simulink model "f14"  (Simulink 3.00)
settings: Solver=ode45  SolverMode=SingleTasking  StartTime=0.0  StopTime=60  RelTol=1e-4  AbsTol=1e-6
PreLoadFcn:
  | f14dat
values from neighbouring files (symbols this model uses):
  a = figure('Color',[0.8 0.8 0.8],     'Position',[25 45 560 420],     'IntegerHandle','off',     'Number','off',    'Name','ÈÎÒâÐÎÊ½×ø±êÑÝÊ¾',    'Tag','Aspectzcx')    [arzcx.m]    (also in f14dat.m = 2.5348; f14def.m = 2.5348; rss.m = zeros([n n arraydims]); watergui.m = 1-str2num(get_param('water/Flush Pulse/PulseConst','value')))
  b = uicontrol('Parent',a,     'Unit',StdUnit,     'BackgroundColor',StdColor,     'Position',PointsPerPixel*[24 28 497 20],     'Units','Normalized',    'Style','text',    'String','Ä¬ÈÏ3DÊÓÍ¼',    'Tag','StatusText')    [arzcx.m]    (also in f14dat.m = 64.13; f14def.m = 64.13; rss.m = b .* (bnz+repmat(zerob,[n m])))
  g = 32.18    [absdata.m]    (also in f14dat.m = 32.2; watergui.m = locdrawwater(hilim, lolim, inflow, outflow, area); watersfun.m = get(ax,'UserData'))
  Ka = 0.6770    (= 0.677)    [f14dat.m]    (also in f14def.m)
  Kf = 1    [absdata.m]    (also in f14dat.m = -1.746; f14def.m = -1.746)
  Ki = -3.8640    (= -3.864)    [f14dat.m]    (also in f14def.m)
  Kq = 0.8156    [f14dat.m]    (also in f14def.m)
  Md = -6.8847    [f14dat.m]    (also in f14def.m)
  Mq = -0.6571    [f14dat.m]    (also in f14def.m)
  Mw = -0.00592    [f14dat.m]    (also in f14def.m)
  Swg = 3    [f14dat.m]    (also in f14def.m)
  Ta = 0.0500    (= 0.05)    [f14dat.m]    (also in f14def.m)
  Tal = 0.3959    [f14dat.m]    (also in f14def.m)
  Ts = 0.1000    (= 0.1)    [f14dat.m]    (also in f14def.m)
  Uo = 689.4000    (= 689.4)    [f14dat.m]    (also in f14def.m)
  Vto = 690.4000    (= 690.4)    [f14dat.m]    (also in f14def.m)
  W1 = 2.9710    (= 2.971)    [f14dat.m]    (also in f14def.m)
  W2 = 4.1440    (= 4.144)    [f14dat.m]    (also in f14def.m)
  Zd = -63.9979    [f14dat.m]    (also in f14def.m)
  Zw = -0.6385    [f14dat.m]    (also in f14def.m)
libraries: simulink x1

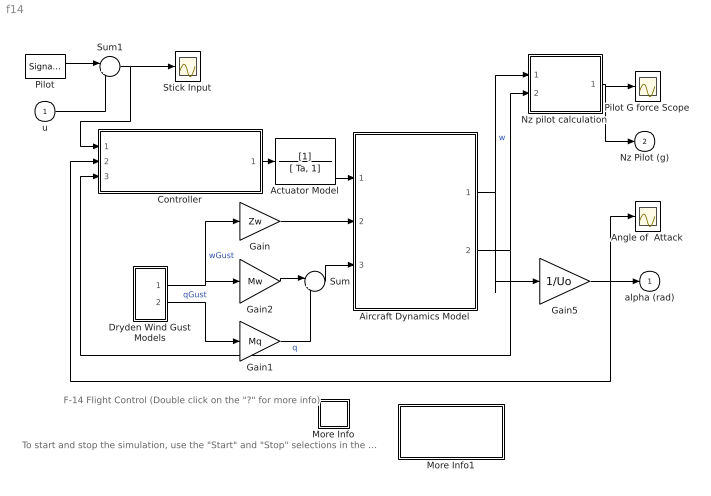
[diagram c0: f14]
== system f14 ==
  note: To start and stop the simulation, use the "Start" and "Stop" selections in the "Simulation" pull-down menu.
  note: F-14 Flight Control (Double click on the "?" for more info)
  u : Inport  Port=1  PortWidth=-1  SampleTime=-1  DataType=auto
  Actuator Model : TransferFcn  Numerator=[1]  Denominator=[ Ta, 1]
  Aircraft Dynamics Model : Subsystem
  Angle of  Attack : Scope
  Controller : Subsystem
  Dryden Wind Gust Models : Subsystem
  Gain : Gain  Gain=Zw  SaturateOnIntegerOverflow=on
  Gain1 : Gain  Gain=Mq  SaturateOnIntegerOverflow=on
  Gain2 : Gain  Gain=Mw  SaturateOnIntegerOverflow=on
  Gain5 : Gain  Gain=1/Uo  SaturateOnIntegerOverflow=on
  More Info : Subsystem
  More Info1 : Subsystem
  Nz pilot calculation : Subsystem
  Pilot : SignalGenerator  WaveForm=square  Amplitude=1  Frequency=0.500000  Units=rad/sec
  Pilot G force Scope : Scope
  Stick Input : Scope
  Sum : Sum  Inputs=|++  SaturateOnIntegerOverflow=on
  Sum1 : Sum  Inputs=|++  SaturateOnIntegerOverflow=on
  alpha (rad) : Outport  Port=1  InitialOutput=0
  Nz Pilot (g) : Outport  Port=2  InitialOutput=0
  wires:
  Gain5/1 -> alpha (rad)/1, Angle of  Attack/1, Controller/2(alpha (rad))
  Aircraft Dynamics Model/1(Vertical Velocity w (ft/sec)) -> Gain5/1, Nz pilot calculation/1(w)  "w"
  Nz pilot calculation/1(Pilot g force (g)) -> Pilot G force Scope/1, Nz Pilot (g)/1
  Gain2/1 -> Sum/1
  Gain/1 -> Aircraft Dynamics Model/2(Vertical Gust wGust (ft/sec))
  Pilot/1 -> Sum1/1
  u/1 -> Sum1/2
  Dryden Wind Gust Models/2(Qg) -> Gain1/1  "qGust"
  Dryden Wind Gust Models/1(Wg) -> Gain2/1, Gain/1  "wGust"
  Sum/1 -> Aircraft Dynamics Model/3(Rotary Gust qGust (rad/sec))
  Gain1/1 -> Sum/2
  Aircraft Dynamics Model/2(Pitch Rate q (rad/sec)) -> Nz pilot calculation/2(q), Controller/3(q (rad/sec))  "q"
  Actuator Model/1 -> Aircraft Dynamics Model/1(Elevator Deflection d (deg))
  Controller/1(Elevator Command (deg)) -> Actuator Model/1
  Sum1/1 -> Stick Input/1, Controller/1(Stick Input (in))

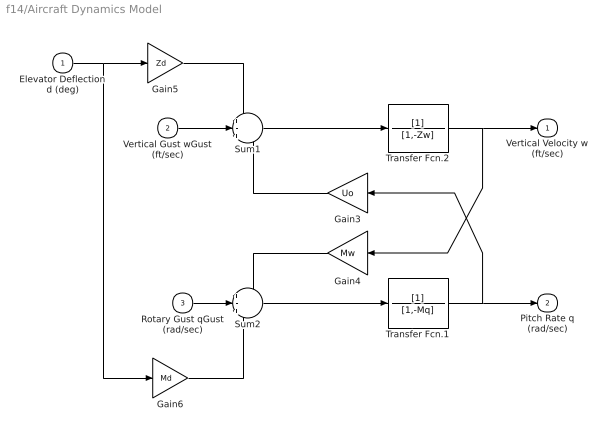
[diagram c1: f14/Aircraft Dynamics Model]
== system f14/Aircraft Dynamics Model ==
  Elevator Deflection d (deg) : Inport  Port=1  PortWidth=-1  SampleTime=-1  DataType=auto
  Vertical Gust wGust (ft/sec) : Inport  Port=2  PortWidth=-1  SampleTime=-1  DataType=auto
  Rotary Gust qGust (rad/sec) : Inport  Port=3  PortWidth=-1  SampleTime=-1  DataType=auto
  Gain3 : Gain  Orientation=left  Gain=Uo  SaturateOnIntegerOverflow=on
  Gain4 : Gain  Orientation=left  Gain=Mw  SaturateOnIntegerOverflow=on
  Gain5 : Gain  Gain=Zd  SaturateOnIntegerOverflow=on
  Gain6 : Gain  Gain=Md  SaturateOnIntegerOverflow=on
  Sum1 : Sum  Inputs=+-+  SaturateOnIntegerOverflow=on
  Sum2 : Sum  Inputs=+-+  SaturateOnIntegerOverflow=on
  Transfer Fcn.1 : TransferFcn  Numerator=[1]  Denominator=[1,-Mq]
  Transfer Fcn.2 : TransferFcn  Numerator=[1]  Denominator=[1,-Zw]
  Vertical Velocity w (ft/sec) : Outport  Port=1  InitialOutput=0
  Pitch Rate q (rad/sec) : Outport  Port=2  InitialOutput=0
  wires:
  Transfer Fcn.2/1 -> Vertical Velocity w (ft/sec)/1, Gain4/1
  Transfer Fcn.1/1 -> Pitch Rate q (rad/sec)/1, Gain3/1
  Gain6/1 -> Sum2/3
  Gain5/1 -> Sum1/1
  Gain3/1 -> Sum1/3
  Rotary Gust qGust (rad/sec)/1 -> Sum2/2
  Sum2/1 -> Transfer Fcn.1/1
  Sum1/1 -> Transfer Fcn.2/1
  Gain4/1 -> Sum2/1
  Vertical Gust wGust (ft/sec)/1 -> Sum1/2
  Elevator Deflection d (deg)/1 -> Gain5/1, Gain6/1

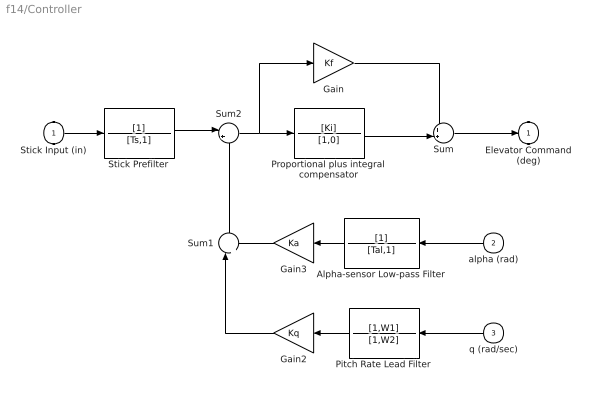
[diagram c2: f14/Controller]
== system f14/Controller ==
  Stick Input (in) : Inport  Port=1  PortWidth=-1  SampleTime=-1  DataType=auto
  alpha (rad) : Inport  Orientation=left  Port=2  PortWidth=-1  SampleTime=-1  DataType=auto
  q (rad/sec) : Inport  Orientation=left  Port=3  PortWidth=-1  SampleTime=-1  DataType=auto
  Alpha-sensor Low-pass Filter : TransferFcn  Orientation=left  Numerator=[1]  Denominator=[Tal,1]
  Gain : Gain  Gain=Kf  SaturateOnIntegerOverflow=on
  Gain2 : Gain  Orientation=left  Gain=Kq  SaturateOnIntegerOverflow=on
  Gain3 : Gain  Orientation=left  Gain=Ka  SaturateOnIntegerOverflow=on
  Pitch Rate Lead Filter : TransferFcn  Orientation=left  Numerator=[1,W1]  Denominator=[1,W2]
  Proportional plus integral compensator : TransferFcn  Numerator=[Ki]  Denominator=[1,0]
  Stick Prefilter : TransferFcn  Numerator=[1]  Denominator=[Ts,1]
  Sum : Sum  Inputs=++|  SaturateOnIntegerOverflow=on
  Sum1 : Sum  Orientation=up  Inputs=|++  SaturateOnIntegerOverflow=on
  Sum2 : Sum  Inputs=|+-  SaturateOnIntegerOverflow=on
  Elevator Command (deg) : Outport  Port=1  InitialOutput=0
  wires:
  Sum2/1 -> Proportional plus integral compensator/1, Gain/1
  Gain/1 -> Sum/1
  Proportional plus integral compensator/1 -> Sum/2
  Stick Prefilter/1 -> Sum2/1
  Sum/1 -> Elevator Command (deg)/1
  Gain2/1 -> Sum1/1
  Gain3/1 -> Sum1/2
  Sum1/1 -> Sum2/2
  Pitch Rate Lead Filter/1 -> Gain2/1
  q (rad/sec)/1 -> Pitch Rate Lead Filter/1
  Alpha-sensor Low-pass Filter/1 -> Gain3/1
  alpha (rad)/1 -> Alpha-sensor Low-pass Filter/1
  Stick Input (in)/1 -> Stick Prefilter/1

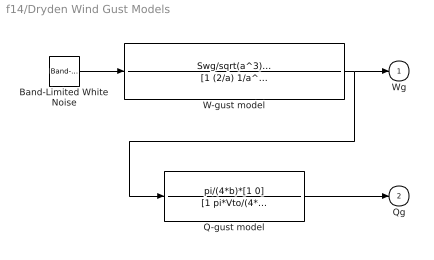
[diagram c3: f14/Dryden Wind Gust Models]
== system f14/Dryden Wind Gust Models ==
  Band-Limited White Noise : simulink/Sources/Band-Limited White Noise  Cov=1  Ts=0.1  seed=[23341]
  Q-gust model : TransferFcn  Numerator=pi/(4*b)*[1 0]  Denominator=[1 pi*Vto/(4*b)]
  W-gust model : TransferFcn  Numerator=Swg/sqrt(a^3)*[sqrt(3)*a,1]  Denominator=[1 (2/a) 1/a^2]
  Wg : Outport  Port=1  InitialOutput=0
  Qg : Outport  Port=2  InitialOutput=0
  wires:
  Band-Limited White Noise/1 -> W-gust model/1
  Q-gust model/1 -> Qg/1
  W-gust model/1 -> Wg/1, Q-gust model/1

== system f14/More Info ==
  note: This demonstration shows a flight controller for the longitudinal motion of a Grumman Aerospace F-14.
  note: Try experimenting with the values in the gain blocks and the signal generators.

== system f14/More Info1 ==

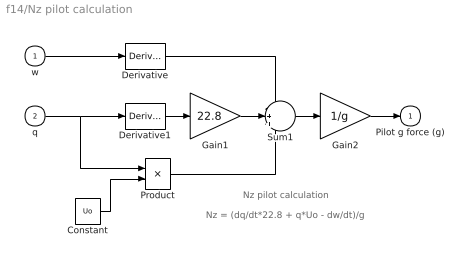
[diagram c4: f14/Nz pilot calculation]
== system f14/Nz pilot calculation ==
  note: Nz pilot calculation
  note: Nz = (dq/dt*22.8 + q*Uo - dw/dt)/g
  w : Inport  Port=1  PortWidth=-1  SampleTime=-1  DataType=auto
  q : Inport  Port=2  PortWidth=-1  SampleTime=-1  DataType=auto
  Constant : Constant  Value=Uo
  Derivative : Derivative
  Derivative1 : Derivative
  Gain1 : Gain  Gain=22.8  SaturateOnIntegerOverflow=on
  Gain2 : Gain  Gain=1/g  SaturateOnIntegerOverflow=on
  Product : Product  Inputs=2  SaturateOnIntegerOverflow=on
  Sum1 : Sum  Inputs=-++  SaturateOnIntegerOverflow=on
  Pilot g force (g) : Outport  Port=1  InitialOutput=0
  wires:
  q/1 -> Product/1, Derivative1/1
  Constant/1 -> Product/2
  Gain2/1 -> Pilot g force (g)/1
  Sum1/1 -> Gain2/1
  Derivative1/1 -> Gain1/1
  Gain1/1 -> Sum1/2
  Product/1 -> Sum1/3
  Derivative/1 -> Sum1/1
  w/1 -> Derivative/1
